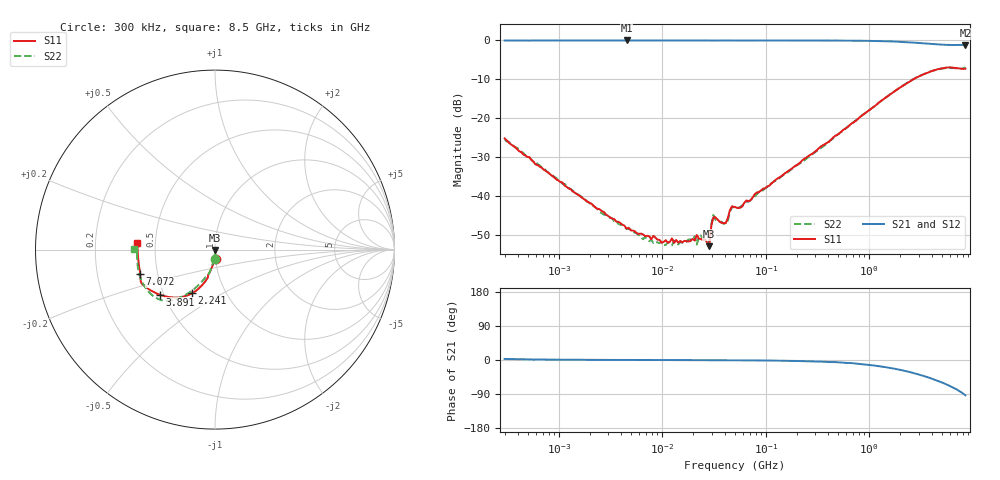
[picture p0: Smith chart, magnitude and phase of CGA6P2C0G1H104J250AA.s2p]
! S-parameter Generated by TDK Corporation
! Copyright(C) 2015 TDK Corporation.
! All Rights Reserved.
! TDK P/N: CGA6P2C0G1H104J250AA (Multilayer Ceramic Chip Capacitors)
! Property: C=100nF
! Size(LxWxT): 3.2x2.5x2.5mm, 0.126x0.098x0.098inches
! Model Type: s2p (Touchstone File Format Version 1.0)
! Frequency: DC=Yes Start=0.3MHz Stop=8500MHz 225points Log-sweep
! Note:
! Model Generated on Jun. 23, 2015
! Hash(MD5):
! Port Assignments:
!  1 ---| |--- 2
! Applicable Conditions:
!  Temperature = 25 degC
!  DC Bias Voltage = 0 V
!  Small Signal Operation
! Terms and conditions regarding TDK Simulation Models
! (1)This simulation model is being provided solely for informational purposes. Please refer to the specifications of the products in terms of detailed characteristics of such products.
! (2)In no event shall TDK Corporation of any of its subsidiaries be liable for any loss or damage arising, directly or indirectly,
!  From any information contained in this simulation model, including, but not limited to loss or damages arising from any inaccuracies, omissions or errors in connection with such information.
! (3)Any and all copyrights on this simulation model are owned by TDK Corporation.
!  Duplication or redistribution of this simulation model without prior written permission from TDK Corporation is prohibited.
! (4)This simulation model is subject to any modification or change without any prior notice.
! (5)Neither TDK Corporation nor any of its subsidiaries shall make any warranty, express or implied,
!  Including but not limited to the correctness, implied warranties of merchantability and fitness for a particular purpose with respect to this simulation models.
! (6)The use of this simulation model shall be deemed to have consented to the terms and conditions hereof.
# MHz S MA R 50
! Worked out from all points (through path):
!   224 points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, 300 kHz to 8.5 GHz, reference 50 ohm
!   highest |S21| = 0.00 dB at 4.519 MHz (marker M1); lowest = -1.3 dB at 8.5 GHz (marker M2)
!   group delay of S21, straight-line fit = 32.2 ps
!   lowest |S11| = -52.9 dB at 28.43 MHz (marker M3), VSWR 1.00, Z = 50.1 - j0.195 ohm
!   |S11| at or under -10 dB: start of sweep to 2.676 GHz
!   |S22| runs from -52.7 to -6.9 dB; largest |S21 - S12| = 0.01
!   S11 on the Smith chart (normalised r, x): 300 kHz: 1.00, -0.11; 2.241 GHz: 0.69, -0.36; 3.891 GHz: 0.48, -0.28; 7.072 GHz: 0.40, -0.14; 8.5 GHz: 0.39, +0.03
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0.3  0.05514 -85.9  0.9984 2.9  0.9951 3.2  0.05396 -88.0
1.72111  0.009301 -85.3  0.9999 0.4  0.9993 0.5  0.009425 -91.5
4.519427  0.003835 -90.4  1 0.1  0.9998 0.1  0.003789 -87.7
9.430415  0.002745 -80.1  0.9999 -0.1  0.9991 -0.0  0.002489 -85.8
14.2633  0.002524 -79.1  0.9995 -0.2  0.9998 -0.2  0.002387 -86.7
20.60362  0.002686 -74.8  0.9996 -0.3  0.9984 -0.3  0.003052 -84.2
21.57293  0.003158 -78.4  0.9983 -0.4  0.9985 -0.4  0.002388 -77.3
23.65048  0.002802 -83.7  0.9999 -0.3  0.9992 -0.3  0.003129 -87.1
28.42509  0.002273 -58.8  0.9993 -0.5  0.9983 -0.5  0.00244 -65.1
29.76236  0.004101 -43.1  0.9962 -0.5  0.9967 -0.5  0.004319 -43.4
31.16253  0.005316 -64.2  0.9974 -0.4  0.9974 -0.3  0.005725 -69.1
39.21571  0.004508 -82.3  0.9997 -0.5  0.999 -0.5  0.004389 -85.1
42.99233  0.005199 -66.2  0.9984 -0.6  0.997 -0.6  0.004815 -68.8
47.13265  0.007405 -74.9  0.9981 -0.6  0.9972 -0.5  0.007168 -75.3
51.67171  0.007165 -81.3  0.9992 -0.7  0.9987 -0.7  0.00702 -84.4
283.1228  0.0352 -92.5  0.9978 -3.7  0.996 -3.6  0.03467 -93.6
1551.304  0.1974 -108.4  0.9742 -20.3  0.9742 -20.2  0.1983 -112.8
2240.89  0.2747 -117.8  0.9534 -29.1  0.9505 -28.9  0.2773 -120.7
3890.506  0.397 -140.7  0.9053 -47.8  0.9042 -47.7  0.3994 -134.3
5126.239  0.44 -152.3  0.8834 -60.0  0.8819 -59.8  0.436 -146.0
7072.242  0.4388 -161.7  0.8761 -78.3  0.8727 -78.2  0.4369 -173.1
8500  0.4347 175.3  0.8643 -93.2  0.8678 -92.8  0.4515 179.6
